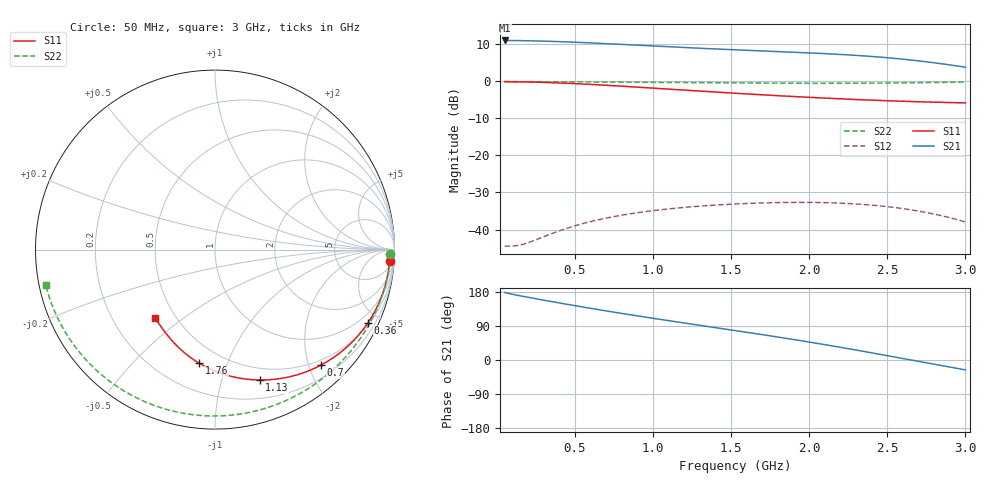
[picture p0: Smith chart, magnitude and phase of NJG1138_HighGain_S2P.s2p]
! NJG1138 High gain mode
# hz S ri R 50
! 2 Port Network Data from SP1.SP block
! freq  reS11  imS11  reS21  imS21  reS12  imS12  reS22  imS22
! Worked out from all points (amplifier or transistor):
!   296 points, 50 MHz to 3 GHz, reference 50 ohm
!   highest |S21| = 10.9 dB at 50 MHz (marker M1)
!   |S21| within 3 dB of that: start of sweep to 1.808 GHz
!   unconditionally stable (mu >= 1): 1.708 GHz to end of sweep
!   at 540 MHz: K = 0.66, MSG = 24.4 dB, |S12| = -38.5 dB
!   at 1.53 GHz: K = 0.93, MSG = 20.7 dB, |S12| = -33.1 dB
!   at 3 GHz: K = 1.62, MAG = 16.2 dB, |S12| = -37.9 dB
!   lowest NFmin = 0.55 dB at 160 MHz
!   S11 on the Smith chart (normalised r, x): 50 MHz: 10, -26; 360 MHz: 0.57, -4.34; 700 MHz: 0.41, -2.21; 1.13 GHz: 0.38, -1.33; 1.76 GHz: 0.37, -0.80; 3 GHz: 0.39, -0.39
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5e7  0.9737 -0.0649  -3.493 0.1152  0.00575 0.00167  0.9773 -0.0239
1.1e8  0.9635 -0.1355  -3.457 0.4513  0.00572 0.00193  0.976 -0.0473
2e8  0.9359 -0.24  -3.352 0.8705  0.00578 0.00332  0.9726 -0.0847
3.6e8  0.8526 -0.4072  -3.036 1.516  0.00676 0.00589  0.9614 -0.1524
4.6e8  0.7835 -0.4947  -2.772 1.855  0.00772 0.00726  0.9511 -0.195
5.5e8  0.714 -0.5608  -2.504 2.112  0.00873 0.00829  0.9397 -0.2337
7e8  0.5898 -0.6438  -2.018 2.443  0.0106 0.0096  0.9159 -0.2991
8.6e8  0.4559 -0.6981  -1.478 2.666  0.0126 0.0104  0.8834 -0.3707
1.04e9  0.3137 -0.7243  -0.88 2.781  0.0149 0.0108  0.836 -0.4548
1.13e9  0.2482 -0.7265  -0.5917 2.793  0.016 0.0107  0.8072 -0.4983
1.33e9  0.1181 -0.7125  0.0141 2.727  0.0183 0.0102  0.7273 -0.5987
1.53e9  0.00995 -0.6807  0.5667 2.552  0.0202 0.00898  0.6194 -0.7019
1.76e9  -0.0893 -0.6323  1.129 2.228  0.0219 0.00688  0.449 -0.815
2.02e9  -0.1739 -0.5717  1.644 1.705  0.0229 0.0036  0.1826 -0.9088
2.15e9  -0.207 -0.5414  1.832 1.385  0.0228 0.00166  0.0195 -0.9268
2.28e9  -0.2352 -0.5121  1.96 1.033  0.0223 -0.000366  -0.159 -0.9149
2.4e9  -0.2574 -0.4863  2.014 0.6918  0.0212 -0.00221  -0.3305 -0.8711
2.51e9  -0.2752 -0.4639  2.004 0.3785  0.0199 -0.00376  -0.4851 -0.8002
2.64e9  -0.2936 -0.4391  1.919 0.0275  0.0178 -0.00527  -0.6531 -0.6789
2.77e9  -0.31 -0.4161  1.762 -0.2804  0.0154 -0.0063  -0.7925 -0.523
2.89e9  -0.3238 -0.3962  1.571 -0.5106  0.013 -0.00674  -0.8872 -0.3582
3e9  -0.3357 -0.379  1.372 -0.6694  0.0108 -0.00671  -0.9427 -0.1993
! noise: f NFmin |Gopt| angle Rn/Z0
5e+07  0.6314  0.854  7.968  0.8983
3.7e+08  0.5744  0.7659  24.14  0.4679
7e+08  0.6635  0.7421  43.52  0.437
1.03e+09  0.7912  0.7164  62.46  0.3971
1.36e+09  0.9467  0.6924  80.44  0.3479
1.68e+09  1.119  0.6724  96.75  0.295
2.01e+09  1.318  0.6546  112.3  0.2393
2.34e+09  1.541  0.6382  126.6  0.1873
2.67e+09  1.792  0.6215  139.6  0.1435
3e+09  2.075  0.6028  151.4  0.1119
